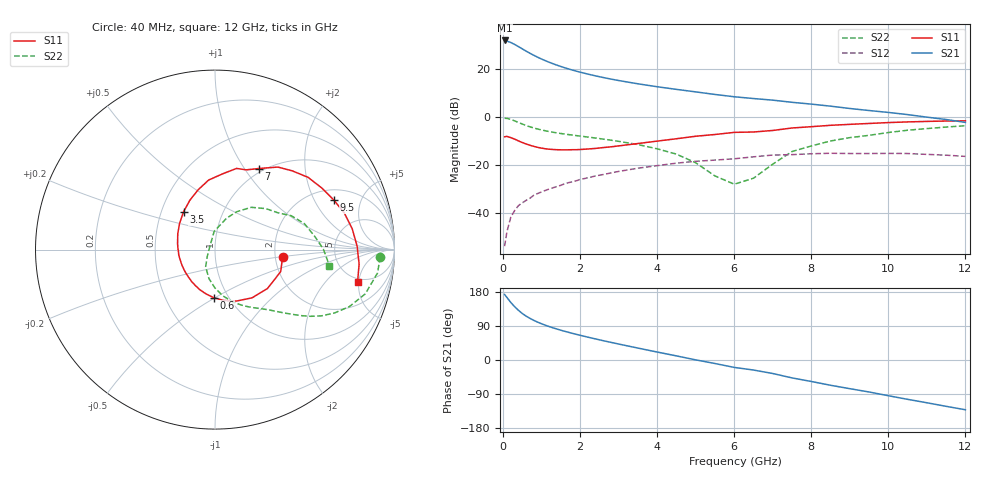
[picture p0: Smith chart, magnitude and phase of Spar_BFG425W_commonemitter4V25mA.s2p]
! Filename: 425bfg425.001
! BFG425W Field C1
! V1=8.370E-001V,V2=4.000E+000V, I1=3.089E-004A, I2=2.505E-002A
# GHz  S  MA  R 50
!  S11  S21  S12  S22
!Freq(GHz)  Mag  Ang  Mag  Ang  Mag  Ang  Mag  Ang
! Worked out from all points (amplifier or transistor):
!   44 points, 40 MHz to 12 GHz, reference 50 ohm
!   highest |S21| = 31.7 dB at 40 MHz (marker M1)
!   |S21| within 3 dB of that: start of sweep to 445.6 MHz
!   unconditionally stable (mu >= 1): start of sweep to 44.69 MHz; 1.233 GHz to end of sweep
!   at 700 MHz: K = 0.81, MSG = 30.2 dB, |S12| = -34.0 dB
!   at 2.4 GHz: K = 1.15, MAG = 18.5 dB, |S12| = -24.7 dB
!   at 12 GHz: K = 1.34, MAG = 3.6 dB, |S12| = -16.6 dB
!   S11 on the Smith chart (normalised r, x): 40 MHz: 2.19, -0.21; 600 MHz: 0.86, -0.49; 3.5 GHz: 0.65, +0.30; 7 GHz: 0.95, +1.16; 9.5 GHz: 2.57, +2.91; 12 GHz: 4.42, -4.83
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0.04  0.379 -6.3  38.41 172.9  0.002 55.9  0.921 -2.5
0.1  0.386 -18.6  37.26 165.0  0.004 77.3  0.915 -8.2
0.2  0.364 -36.6  34.87 151.9  0.008 73.4  0.873 -16.4
0.3  0.339 -52.4  31.75 140.8  0.011 70.1  0.813 -23.0
0.4  0.311 -67.1  28.57 131.1  0.014 67.7  0.752 -28.1
0.5  0.288 -80.2  25.63 122.5  0.016 65.6  0.698 -31.9
0.6  0.268 -91.4  22.99 115.7  0.018 64.2  0.65 -34.9
0.7  0.252 -101.4  20.74 109.8  0.02 63.2  0.61 -37.2
0.9  0.228 -118.9  17.17 99.8  0.025 61.8  0.549 -40.7
1.2  0.209 -140.0  13.48 88.1  0.031 60.0  0.487 -45.1
1.6  0.202 -162.7  10.38 75.7  0.04 57.3  0.432 -50.3
2.2  0.211 171.1  7.656 60.3  0.053 51.7  0.374 -58.9
2.8  0.234 149.9  6.03 46.5  0.067 44.8  0.322 -68.3
3.5  0.274 129.8  4.806 31.5  0.084 35.5  0.261 -80.5
4.5  0.345 106.1  3.68 10.8  0.107 20.8  0.165 -101.8
5.5  0.423 84.6  2.885 -9.3  0.124 5.2  0.058 -138.3
6.5  0.477 68.6  2.372 -26.5  0.145 -7.0  0.052 112.6
7  0.513 61.7  2.195 -35.6  0.158 -14.7  0.102 92.5
8.5  0.657 37.7  1.646 -66.7  0.172 -44.1  0.31 49.5
9.5  0.718 22.5  1.335 -84.4  0.17 -60.8  0.406 30.3
10.5  0.773 8.7  1.098 -103.8  0.17 -79.5  0.519 16.1
12  0.815 -13.0  0.755 -131.3  0.148 -109.5  0.644 -8.0
